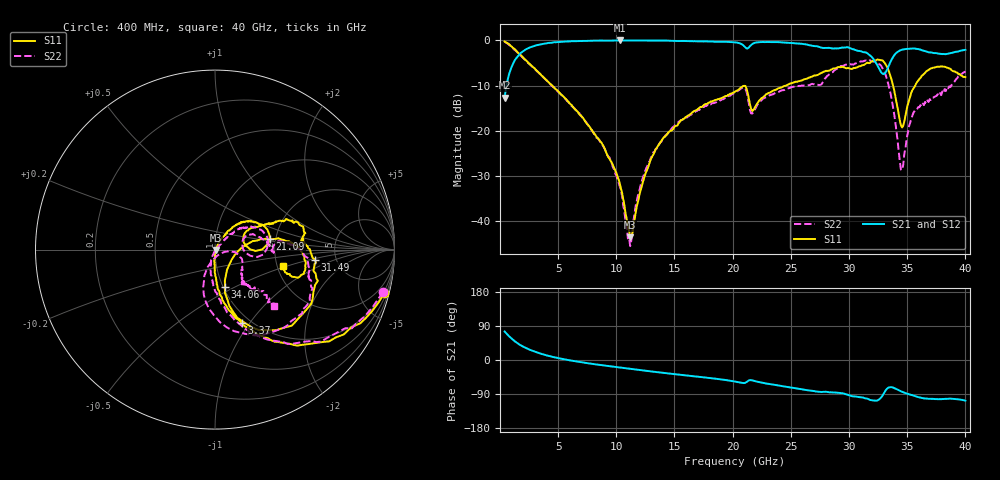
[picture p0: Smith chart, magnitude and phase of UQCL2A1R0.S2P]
! AVX Corporation
! Date:  10/27/06
! Part No:  UQCL2A1R0
! Description:  Ultra Low ESR Microwave capacitors
! Mounting Orientation:  Horizontal
# GHZ S DB R 50
! Freq  |S11|  S11 Ph  |S21|  S21 Ph  |S12|  S12 Ph  |S22|  S22 Ph
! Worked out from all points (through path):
!   401 points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, 400 MHz to 40 GHz, reference 50 ohm
!   highest |S21| = 0.00 dB at 10.3 GHz (marker M1); lowest = -12.7 dB at 400 MHz (marker M2)
!   group delay of S21, straight-line fit = 10 ps
!   lowest |S11| = -43.6 dB at 11.19 GHz (marker M3), VSWR 1.01, Z = 50.6 - j0.228 ohm
!   |S11| at or under -10 dB: 4.494 GHz to 24.59 GHz (20.1 GHz wide, 138 % of centre); 33.78 GHz to 35.68 GHz (1.903 GHz wide, 5.48 % of centre)
!   |S22| runs from -45.6 to -0.3 dB; largest |S21 - S12| = 0.024
!   S11 on the Smith chart (normalised r, x): 400 MHz: 0.83, -7.80; 3.37 GHz: 0.91, -0.92; 21.09 GHz: 1.86, +0.25; 31.49 GHz: 3.44, -0.55; 34.06 GHz: 1.02, -0.45; 40 GHz: 2.16, -0.48
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0.4  -0.23 -14.5  -12.70 75.2  -12.78 75.2  -0.31 -14.3
1.39  -2.26 -42.3  -3.97 46.8  -3.97 47.1  -2.33 -42.4
3.37  -7.20 -70.0  -0.95 18.1  -0.92 18.3  -7.28 -72.1
7.033  -16.92 -89.2  -0.13 -6.1  -0.07 -6.1  -16.87 -99.1
8.914  -23.49 -93.1  -0.04 -14.6  -0.02 -14.7  -23.64 -109.0
10.3  -31.74 -89.0  0.00 -19.9  -0.01 -20.2  -32.36 -110.6
11.191  -43.64 -20.0  -0.01 -23.2  -0.01 -23.5  -45.62 -21.9
12.28  -31.45 59.8  -0.01 -27.5  -0.01 -27.7  -30.42 42.5
13.666  -23.07 59.7  -0.02 -32.5  0.00 -32.8  -23.12 45.6
20.2  -11.35 34.6  -0.42 -56.7  -0.50 -56.4  -11.67 26.2
21.091  -10.09 11.2  -1.54 -60.0  -1.61 -59.6  -10.76 1.2
21.784  -15.45 21.3  -0.64 -54.5  -0.70 -54.3  -15.95 16.5
26.833  -8.01 23.9  -1.18 -81.1  -1.18 -81.5  -9.61 -2.6
28.615  -6.23 18.0  -1.77 -85.5  -1.81 -86.0  -7.01 1.1
31.486  -5.05 -5.7  -2.70 -101.5  -2.73 -101.4  -4.44 -29.7
32.674  -4.35 -35.8  -6.67 -101.7  -6.67 -101.6  -5.39 -63.0
33.466  -7.15 -68.0  -5.30 -72.1  -5.30 -71.9  -10.63 -100.1
34.06  -13.34 -74.8  -2.77 -76.5  -2.78 -76.4  -19.73 -112.7
34.555  -19.28 -32.0  -2.05 -83.8  -2.07 -83.6  -28.77 -43.4
35.545  -10.61 12.1  -1.78 -93.8  -1.80 -93.5  -15.98 -18.9
36.832  -6.53 0.7  -2.62 -102.3  -2.55 -101.6  -13.65 -44.8
40  -8.13 -13.8  -2.06 -107.3  -1.99 -106.4  -6.87 -43.8
